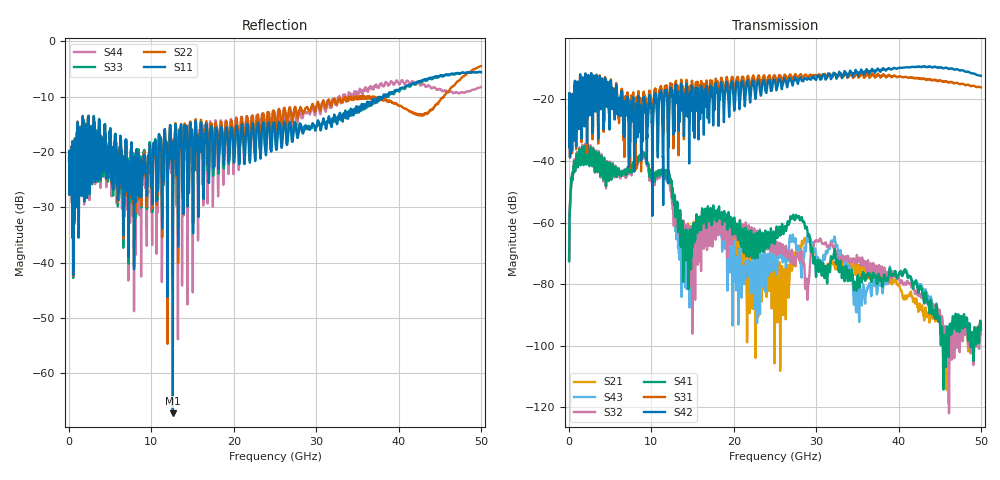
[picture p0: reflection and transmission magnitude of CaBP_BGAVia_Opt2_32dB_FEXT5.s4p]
!* Samtec Inc. NovaRay Examax Flyover System  *
!*  REV DATE  = 08/08/18  *
!*  TYPE  = TOUCHSTONE  *
!*  PORTS  = 4 port  *
!*  UNITS  = GHz  *
!*  DATA RANGE = DC  to 50 GHz; 10 MHz Step  *
!*  PARAMETER  = S  *
!*  FORMAT  = Real-Imaginary  *
!*  REFERENCE  = 50 ohms  *
!*  SOURCE  = HFSS  *
!*  VALIDATED  = No  *
!*  MANUFACTURER = SAMTEC  *
!*  INTERCONNECT = NVAx to EBCx to EBCx to NVAx  *
!*  [Full Channel NVAx to EBCx to EBCx to NVAx  with PCB Trace and BGA Via]  *
!*  BOUNDARY A  = Silicon BGA Ball Pad  *
!*  BOUNDARY B  = Silicon BGA Ball Pad  *
!*  NVAx (end a) ->>- (end b) NVAx  *
!*  Port 01 ->>- Port 02  *
!*  Port 03 ->>- Port 04  *
!***************************** CHANNEL MODEL ******************************************
# GHz S RI R 50
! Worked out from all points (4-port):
!   5000 points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, 10 MHz to 50 GHz, reference 50 ohm
!   strongest paths, dB at 10 MHz, 12.51 GHz, 25.01 GHz, 37.51 GHz, 50 GHz:
!     S42: -23.1, -16.9, -13.9, -10.1, -12.4
!     S31: -23.1, -15.2, -12.2, -11.7, -16.1
!     S41: -72.5, -50.3, -66.0, -78.4, -94.7
!     S32: -71.9, -54.0, -67.2, -76.6, -96.2
!     S43: -72.1, -52.8, -73.5, -80.0, -96.3
!     S21: -72.3, -51.9, -77.0, -76.9, -94.9
!   lowest |S11| = -67.2 dB at 12.6 GHz (marker M1), VSWR 1.00, Z = 50 + j0.0147 ohm
!   |S11| at or under -10 dB: start of sweep to 37.74 GHz; 37.74 GHz to 38.13 GHz (385.5 MHz wide, 1.02 % of centre); 38.51568 GHz to 38.54961 GHz (33.93 MHz wide, 0.0881 % of centre)
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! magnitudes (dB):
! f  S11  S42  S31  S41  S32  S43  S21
! 10 MHz  -21.6  -23.1  -23.1  -72.5  -71.9  -72.1  -72.3
! 1.42 GHz  -16.7  -13.5  -13.7  -40.3  -39.7  -39.9  -40.0
! 12.6 GHz  -67.2  -22.6  -21.8  -52.1  -55.7  -55.6  -53.8
! 14.76 GHz  -15.5  -17.9  -15.7  -64.2  -64.1  -70.2  -63.5
! 16.33 GHz  -27.5  -24.2  -19.0  -59.7  -65.4  -61.8  -63.3
! 20.4 GHz  -15.8  -14.3  -12.9  -60.4  -60.4  -71.0  -61.8
! 50 GHz  -5.5  -12.4  -16.1  -94.7  -96.2  -96.3  -94.9
